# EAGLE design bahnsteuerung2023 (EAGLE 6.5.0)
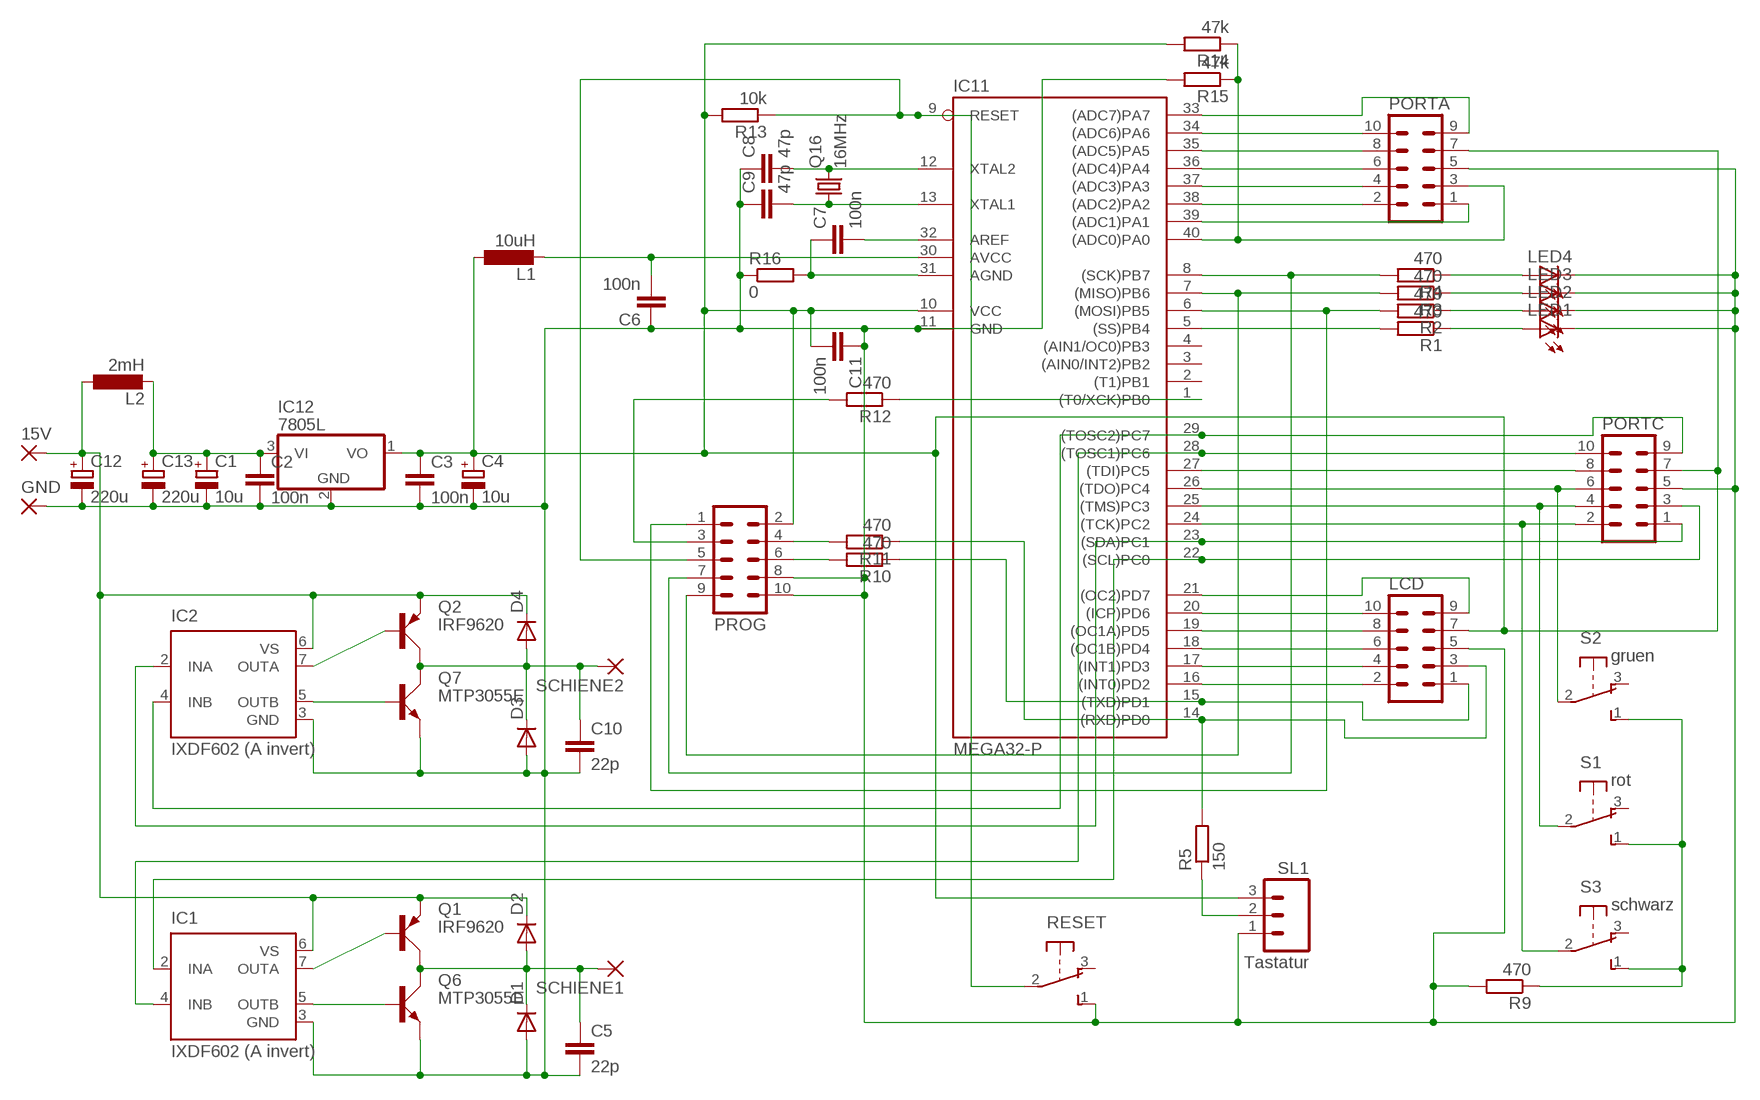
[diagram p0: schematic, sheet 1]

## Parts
15V  1,6/0,8  [1,6/0,8]
C1  10u  CPOL-EUE2.5-5  [E2,5-5]
C2  100n  C5/2.5  [C5B2.5]
C3  100n  C5/2.5  [C5B2.5]
C4  10u  CPOL-EUE2.5-5  [E2,5-5]
C5  22p  C2.5/2  [C2.5-2]
C6  100n  C5/2.5  [C5B2.5]
C7  100n  C2.5/2  [C2.5-2]
C8  47p  C2.5/2  [C2.5-2]
C9  47p  C2.5/2  [C2.5-2]
C10  22p  C2.5/2  [C2.5-2]
C11  100n  C2.5/2  [C2.5-2]
C12  220u  CPOL-EUE2.5-5  [E2,5-5]
C13  220u  CPOL-EUE2.5-5  [E2,5-5]
D1  1N4148DO35-10  [DO35-10]
D2  1N4148DO35-10  [DO35-10]
D3  1N4148DO35-10  [DO35-10]
D4  1N4148DO35-10  [DO35-10]
GND  1,6/0,8  [1,6/0,8]
IC1  IXDF602 (A invert)  IR4427S  [SO08]
IC2  IXDF602 (A invert)  IR4427S  [SO08]
IC11  MEGA32-P  [DIL40]
IC12  7805L  [TO92]
L1  10uH  L-EU0204/7  [0204/7@1]
L2  2mH  L-EU0204/7  [0204/7@1]
LCD  ML10  [ML10]
LED1  LED3MM  [LED3MM]
LED2  LED3MM  [LED3MM]
LED3  LED3MM  [LED3MM]
LED4  LED3MM  [LED3MM]
PORTA  ML10  [ML10]
PORTC  ML10  [ML10]
PROG  ML10  [ML10]
Q1  IRF9620  MJE2955  [TO220AV@1]
Q2  IRF9620  MJE2955  [TO220AV@1]
Q6  MTP3055E  MJE3055  [TO220AV]
Q7  MTP3055E  MJE3055  [TO220AV]
Q16  16MHz  CRYTALHC49U-V  [HC49U-V]
R1  470  R-EU_0204/7  [0204/7]
R2  470  R-EU_0204/7  [0204/7]
R3  470  R-EU_0204/7  [0204/7]
R4  470  R-EU_0204/7  [0204/7]
R5  150  R-EU_0204/7  [0204/7]
R9  470  R-EU_0204/7  [0204/7]
R10  470  R-EU_0204/7  [0204/7]
R11  470  R-EU_0204/7  [0204/7]
R12  470  R-EU_0204/7  [0204/7]
R13  10k  R-EU_0204/7  [0204/7]
R14  47k  R-EU_0204/7  [0204/7]
R15  47k  R-EU_0204/7  [0204/7]
R16  0  R-EU_0204/2V  [0204V]
RESET  9077-1  [9077-1]
S1  rot  9077-1  [9077-1]
S2  gruen  9077-1  [9077-1]
S3  schwarz  9077-1  [9077-1]
SCHIENE1  1,6/0,8  [1,6/0,8]
SCHIENE2  1,6/0,8  [1,6/0,8]
SL1  Tastatur  M03  [03P]

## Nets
AGND [mitteldick]: C7.1 IC11.31(AGND) R16.2
AREF [mitteldick]: C7.2 IC11.32(AREF)
AVCC [mitteldick]: C6.2 IC11.30(AVCC) L1.2
GND [mitteldick]: C1.- C2.2 C3.2 C4.- C5.2 C6.1 C8.1 C9.1 C10.2 C11.1 C12.- C13.- D1.A D3.A GND.1(P) IC1.3(GND) IC2.3(GND) IC11.11(GND) IC12.2(GND) LCD.5 LED1.K(C) LED2.K(C) LED3.K(C) LED4.K(C) PORTA.5 PORTC.5 PROG.8 PROG.10 Q6.E Q7.E R9.2 R15.2 R16.1 RESET.1(S) SL1.1
N$1: IC1.2(INA) IC11.22((SCL)PC0) PORTC.3
N$2: IC2.2(INA) IC11.23((SDA)PC1) PORTC.1
N$3: IC11.24((TCK)PC2) PORTC.2 S3.2(P)
N$4: IC11.25((TMS)PC3) PORTC.4 S1.2(P)
N$5 [mitteldick]: IC2.5(OUTB) Q7.B
N$6: IC11.5((SS)PB4) R1.2
N$7: LED1.A R1.1
N$8: LED2.A R2.1
N$9: LED3.A R3.1
N$10: LED4.A R4.1
N$11 [mitteldick]: IC11.16((INT0)PD2) LCD.2
N$12 [mitteldick]: IC11.17((INT1)PD3) LCD.4
N$13 [mitteldick]: IC11.18((OC1B)PD4) LCD.6
N$14 [mitteldick]: IC11.19((OC1A)PD5) LCD.8
N$15 [mitteldick]: IC11.20((ICP)PD6) LCD.10
N$16 [mitteldick]: IC11.21((OC2)PD7) LCD.9
N$17 [mitteldick]: IC1.5(OUTB) Q6.B
N$18 [mitteldick]: IC11.26((TDO)PC4) PORTC.6 S2.2(P)
N$19 [mitteldick]: IC11.27((TDI)PC5) PORTC.8
N$20 [mitteldick]: IC1.4(INB) IC11.28((TOSC1)PC6) PORTC.10
N$21 [mitteldick]: IC2.4(INB) IC11.29((TOSC2)PC7) PORTC.9
N$22 [mitteldick]: IC11.39((ADC1)PA1) PORTA.1
N$23 [mitteldick]: IC11.38((ADC2)PA2) PORTA.2
N$24 [mitteldick]: IC11.37((ADC3)PA3) PORTA.4
N$25 [mitteldick]: IC11.36((ADC4)PA4) PORTA.6
N$26 [mitteldick]: IC11.35((ADC5)PA5) PORTA.8
N$27 [mitteldick]: IC11.34((ADC6)PA6) PORTA.10
N$28 [mitteldick]: IC11.33((ADC7)PA7) PORTA.9
N$29 [mitteldick]: R9.1 S1.1(S) S2.1(S) S3.1(S)
N$30: R5.1 SL1.2
N$31 [mitteldick]: C1.+ C2.1 C13.+ IC12.3(VI) L2.2
N$32: C5.1 D1.C D2.A Q1.C Q6.C SCHIENE1.1(P)
N$34: IC1.7(OUTA) Q1.B
N$35: C10.1 D3.C D4.A Q2.C Q7.C SCHIENE2.1(P)
N$37: IC2.7(OUTA) Q2.B
N$122: IC11.40((ADC0)PA0) PORTA.3 R14.1 R15.1
N$135: IC11.6((MOSI)PB5) PROG.1 R2.2
N$136: IC11.7((MISO)PB6) PROG.9 R3.2
N$147: IC11.14((RXD)PD0) LCD.3 R5.2 R11.1
N$150: IC11.1((T0/XCK)PB0) R12.1
N$152: C8.2 IC11.12(XTAL2) Q16.2
N$153: C9.2 IC11.13(XTAL1) Q16.1
N$156: IC11.9(RESET) PROG.5 R13.1 RESET.2(P)
N$157: PROG.4 R11.2
N$158: PROG.6 R10.2
N$159: PROG.3 R12.2
N$161: IC11.15((TXD)PD1) LCD.1 R10.1
N$170: IC11.8((SCK)PB7) PROG.7 R4.2
VCC [mitteldick]: C3.1 C4.+ C11.2 IC11.10(VCC) IC12.1(VO) L1.1 LCD.7 PORTA.7 PORTC.7 PROG.2 R13.2 R14.2 SL1.3
VS [mitteldick]: 15V.1(P) C12.+ D2.C D4.C IC1.6(VS) IC2.6(VS) L2.1 Q1.E Q2.E
Unconnected: IC11.2((T1)PB1) IC11.3((AIN0/INT2)PB2) IC11.4((AIN1/OC0)PB3) RESET.3(O) S1.3(O) S2.3(O) S3.3(O)

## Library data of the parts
15V GND SCHIENE1 SCHIENE2 = wirepad:1,6/0,8: THROUGH-HOLE PAD
C1 C4 C12 C13 = rcl:CPOL-EU: POLARIZED CAPACITOR, European symbol
C2 C3 C5-C11 = capacitor-wima:C: CAPACITOR
D1-D4 = diode:1N4148: DIODE
IC1 IC2 = ir:IR4427: DUAL LOW SIDE DRIVER Source: ID4426.pdf; MF: INTERNATIONAL RECTIFIER(IR); MPN: IR4427STRPBF; OC_FARNELL: 8639094; OC_NEWARK: 63J7933
IC11 = atmel:MEGA32-P: MICROCONTROLLER 32 Kbytes FLASH 2 Kbytes SRAM 1 Kbytes EEPROM USART 8-channel 10 bit ADC Source: www.atmel.com .. doc2503.pdf
IC12 = linear:78*: Positive VOLTAGE REGULATOR Source: http://cache.national.com/ds/LM/LM78L05.pdf http://www.fairchildsemi.com/ds/LM/LM7805.pdf
L1 L2 = rcl:L-EU: INDUCTOR, European symbol
LCD PORTA PORTC PROG = con-harting-ml:ML10: HARTING
LED1-LED4 = led:LED: LED
Q1 Q2 = transistor-power:MJE2955: PNP TRANSISTOR
Q6 Q7 = transistor-power:MJE3055: NPN TRANSISTOR
Q16 = crystal:CRYTAL: CRYSTAL
R1-R5 R9-R16 = rcl:R-EU_: RESISTOR, European symbol
RESET S1-S3 = switch-misc:9077-1: MARQUARDT SWITCH
SL1 = con-amp-quick:M03: AMP QUICK CONNECTOR; OC_FARNELL: unknown; OC_NEWARK: unknown

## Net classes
1 dick: width 1.016 mm, clearance 0.61 mm
2 mitteldick: width 0.762 mm

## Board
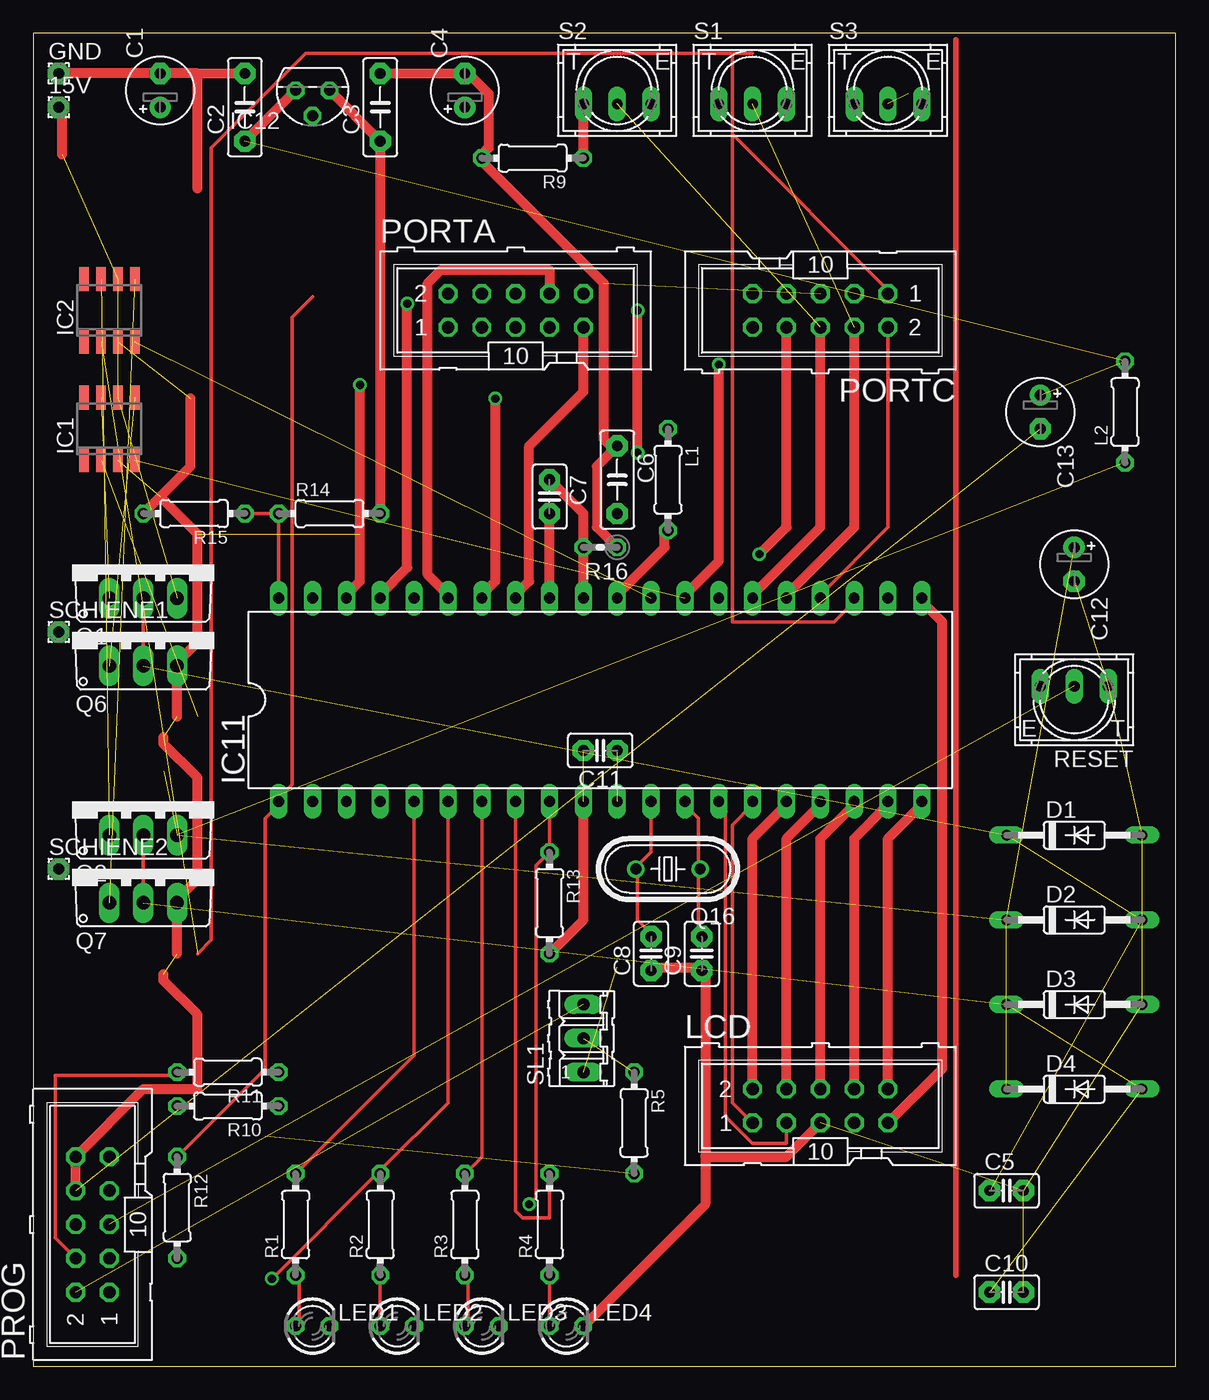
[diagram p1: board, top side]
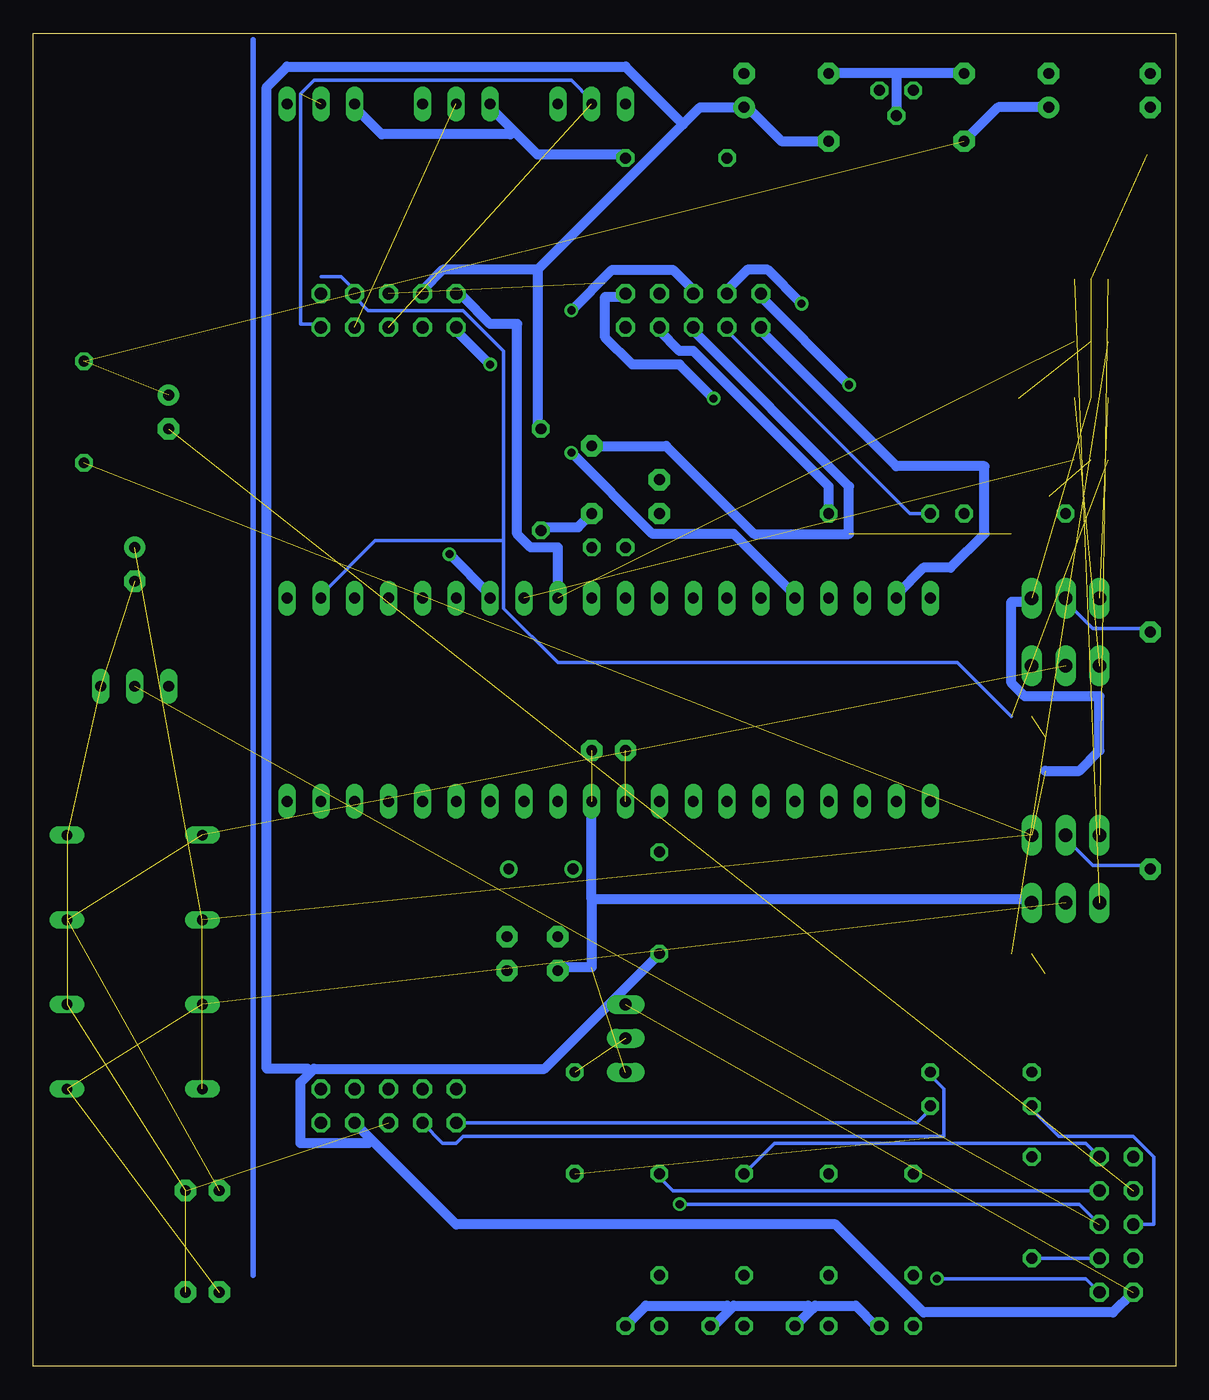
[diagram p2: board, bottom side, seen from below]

Size 85.7 x 100 mm. Coordinates in mm from the lower left corner, seen from the top.
Outline: 0,0 85.7,0 85.7,100 0,100 0,0
Copper layers (1*16): Top 0.035mm / dielectric 1.5mm / Bottom 0.035mm
Design rules "default": minimum track width 10mil, minimum drill 24mil, track to track 8mil, track to pad 8mil, pad to pad 8mil, via to via 8mil, smd to smd 8mil, copper to edge 40mil, drill to drill 8mil, minimum pad ring 10mil, minimum via ring 8mil, stop-mask expansion 4mil, vias tented up to drill 0mil, thermal gap 10mil

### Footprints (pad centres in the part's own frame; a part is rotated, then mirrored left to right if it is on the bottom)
1,6/0,8 = drill 0.813 pad 1.6 octagon: 1 0,0
E2,5-5 = drill 0.813 pad 1.6: + -1.27,0 | drill 0.813 pad 1.6 octagon: - 1.27,0
C5B2.5 = drill 0.813 pad 1.6 octagon: 1 -2.54,0; 2 2.54,0
C2.5-2 = drill 0.813 pad 1.6 octagon: 1 -1.27,0; 2 1.27,0
DO35-10 = drill 0.813 long: A 5.08,0; C -5.08,0
SO08 = smd 0.72 x 1.78: 1 -1.905,-2.35; 2 -0.635,-2.35; 3 0.635,-2.35; 4 1.905,-2.35; 5 1.905,2.35; 6 0.635,2.35; 7 -0.635,2.35; 8 -1.905,2.35
DIL40 = drill 0.813 long: 1 -24.13,-7.62; 2 -21.59,-7.62; 3 -19.05,-7.62; 4 -16.51,-7.62; 5 -13.97,-7.62; 6 -11.43,-7.62; 7 -8.89,-7.62; 8 -6.35,-7.62; 9 -3.81,-7.62; 10 -1.27,-7.62; 11 1.27,-7.62; 12 3.81,-7.62; 13 6.35,-7.62; 14 8.89,-7.62; 15 11.43,-7.62; 16 13.97,-7.62; 17 16.51,-7.62; 18 19.05,-7.62; 19 21.59,-7.62; 20 24.13,-7.62; 21 24.13,7.62; 22 21.59,7.62; 23 19.05,7.62; 24 16.51,7.62; 25 13.97,7.62; 26 11.43,7.62; 27 8.89,7.62; 28 6.35,7.62; 29 3.81,7.62; 30 1.27,7.62; 31 -1.27,7.62; 32 -3.81,7.62; 33 -6.35,7.62; 34 -8.89,7.62; 35 -11.43,7.62; 36 -13.97,7.62; 37 -16.51,7.62; 38 -19.05,7.62; 39 -21.59,7.62; 40 -24.13,7.62
TO92 = drill 0.813 octagon: 1 -1.27,0; 2 0,1.905; 3 1.27,0
0204/7@1 = drill 0.813 octagon: 1 -3.81,0; 2 3.81,0
ML10 = drill 0.914 octagon: 1 -5.08,-1.27; 2 -5.08,1.27; 3 -2.54,-1.27; 4 -2.54,1.27; 5 0,-1.27; 6 0,1.27; 7 2.54,-1.27; 8 2.54,1.27; 9 5.08,-1.27; 10 5.08,1.27
LED3MM = drill 0.813 octagon: A -1.27,0; K 1.27,0
TO220AV@1 = drill 1.016 long: B -2.54,-2.54; C 0,-2.54; E 2.54,-2.54
TO220AV = drill 1.016 long: B -2.54,-2.54; C 0,-2.54; E 2.54,-2.54
HC49U-V = drill 0.813: 1 -2.413,0; 2 2.413,0
0204/7 = drill 0.813 octagon: 1 -3.81,0; 2 3.81,0
0204V = drill 0.813 octagon: 1 -1.27,0; 2 1.27,0
9077-1 = drill 0.813 long: 1 -2.54,-1.016; 2 0,-1.016; 3 2.54,-1.016
03P = drill 0.914 long: 1 -2.54,0; 2 0,0; 3 2.54,0

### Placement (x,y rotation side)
15V  1.9,94.45 0 top
C1  9.52,95.72 90 top
C2  15.87,94.45 90 top
C3  26.03,94.45 90 top
C4  32.38,95.72 90 top
C5  73.02,13.17 0 top
C6  43.81,66.51 270 top
C7  38.73,65.24 270 top
C8  46.35,30.95 90 top
C9  50.16,30.95 90 top
C10  73.02,5.55 0 top
C11  42.54,46.19 180 top
C12  78.1,60.16 270 top
C13  75.56,71.59 270 top
D1  78.1,39.84 0 top
D2  78.1,33.49 0 top
D3  78.1,27.14 0 top
D4  78.1,20.79 0 top
GND  1.9,96.99 0 top
IC1  5.71,70.32 0 top
IC2  5.71,79.21 0 top
IC11  42.54,50 0 top
IC12  20.95,95.72 180 top
L1  47.62,66.51 270 top
L2  81.91,71.59 90 top
LCD  59.05,19.52 0 top
LED1  20.95,3.01 0 top
LED2  27.3,3.01 0 top
LED3  33.65,3.01 0 top
LED4  40,3.01 0 top
PORTA  36.19,79.21 0 top
PORTC  59.05,79.21 180 top
PROG  4.44,10.63 90 top
Q1  8.25,60.16 0 top
Q2  8.25,42.38 0 top
Q6  8.25,55.08 0 top
Q7  8.25,37.3 0 top
Q16  47.62,37.3 180 top
R1  19.68,10.63 90 top
R2  26.03,10.63 90 top
R3  32.38,10.63 90 top
R4  38.73,10.63 90 top
R5  45.08,18.25 270 top
R9  37.46,90.64 180 top
R10  14.6,19.52 180 top
R11  14.6,22.06 180 top
R12  10.79,11.9 270 top
R13  38.73,34.76 270 top
R14  22.22,63.97 0 top
R15  12.06,63.97 180 top
R16  42.54,61.43 180 top
RESET  78.1,50 180 top
S1  53.97,95.72 0 top
S2  43.81,95.72 0 top
S3  64.13,95.72 0 top
SCHIENE1  1.9,55.08 0 top
SCHIENE2  1.9,37.3 0 top
SL1  41.27,24.6 90 top

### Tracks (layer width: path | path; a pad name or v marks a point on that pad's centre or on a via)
AGND
  Top 0.762: IC11.31 R16.2 41.27,63.97 C7.1
AREF
  Top 0.762: IC11.32 C7.2
AVCC
  Top 0.762: IC11.30 43.81,57.87 47.37,61.43 47.37,62.45 L1.2
  Bottom 0.762: C6.2 44.83,62.95 47.37,62.95 L1.2
GND  (15 unrouted)
  Top 0.762: R16.1 42.29,62.95 42.29,67.53 C6.1 43.3,69.05 42.79,69.56 42.79,81.24 33.65,90.39 R9.2 33.65,90.89 34.16,91.4 34.16,95.47 32.63,96.99 C4.- C3.2 | GND.1 C1.- 12.31,96.99 | 12.31,96.99 C2.2 | LCD.5 56.51,15.71 50.41,15.71 | 50.41,15.71 50.41,29.43 C9.1 49.91,29.93 46.35,29.93 C8.1 | LED4.K 50.41,12.15 50.41,15.71 | PROG.8 PROG.10 8.25,20.79 12.31,20.79 12.31,26.38 9.77,28.92 9.77,29.43 | 10.79,30.95 Q7.E 10.79,35.01 12.31,36.54 12.31,44.16 9.77,46.7 9.77,47.21 | 10.79,48.73 Q6.E 10.79,52.79 12.31,54.32 12.31,62.45 9.52,65.24 | 9.52,65.24 11.81,67.53 11.81,72.61 | 9.52,65.24 R15.2 | 12.31,88.35 12.31,96.99
  Bottom 0.762: C6.1 38.22,69.05 31.62,62.45 24.51,62.45 24.51,66 36.19,77.69 PORTA.5 | C2.2 20.95,96.99 | 20.95,96.99 IC12.2 | 20.95,96.99 C3.2 | 27.3,4.28 LED2.K | 27.3,4.28 27.05,4.53 24,4.53 22.47,3.01 LED1.K | 33.4,4.28 33.14,4.53 27.55,4.53 27.3,4.28 | 33.4,4.28 34.67,3.01 LED3.K | LED4.K 39.75,4.53 33.65,4.53 33.4,4.28 | 43.81,35.01 43.81,29.93 46.35,29.93 C8.1 | 43.81,35.01 IC11.11 | 43.81,35.01 10.79,35.01 Q7.E
N$1  (1 unrouted)
  Bottom 0.254: 64.13,81.75 62.61,81.75 61.59,80.73 PORTC.3 61.59,80.23 60.57,79.21 53.46,79.21 50.41,76.16 50.41,61.94 | 12.31,48.73 16.38,52.79 46.35,52.79 50.41,56.86 50.41,61.94 | 50.41,61.94 60.07,61.94 64.13,57.87 IC11.22
N$2  (1 unrouted)
  Top 0.254: 12.31,30.95 13.33,31.97 13.33,91.4 20.44,98.51 52.45,98.51 | 52.45,98.51 53.97,98.51 | 52.45,98.51 52.45,92.42 | 52.45,92.42 52.45,55.84 60.07,55.84 61.59,57.37 IC11.23 | 52.45,92.42 64.13,80.73 PORTC.1
N$3  (1 unrouted)
  Top 0.254: IC11.24 59.05,57.87 64.13,62.95 PORTC.2
  Bottom 0.254: 43.81,94.96 45.33,96.48 64.64,96.48 65.65,95.47 65.65,78.19 64.13,78.19 PORTC.2
N$4  (1 unrouted)
  Top 0.762: IC11.25 56.51,57.87 61.59,62.95 PORTC.4
N$5  (1 unrouted)
N$6
  Top 0.254: R1.2 28.57,23.33 IC11.5
N$7
  Top 0.254: LED1.A 19.93,3.01 19.93,6.57 R1.1
N$8
  Top 0.254: LED2.A R2.1
N$9
  Top 0.254: LED3.A 32.63,3.01 32.63,6.57 R3.1
N$10
  Top 0.254: LED4.A R4.1
N$11
  Top 0.762: LCD.2 53.97,39.59 56.51,42.13 IC11.16
N$12
  Top 0.762: LCD.4 56.51,39.59 59.05,42.13 IC11.17
N$13
  Top 0.762: LCD.6 59.05,39.59 61.59,42.13 IC11.18
N$14
  Top 0.762: LCD.8 61.59,39.59 64.13,42.13 IC11.19
N$15
  Top 0.762: LCD.10 64.13,39.59 66.67,42.13 IC11.20
N$16
  Top 0.762: LCD.9 68.19,22.31 68.19,55.84 66.67,57.37 IC11.21
N$17  (1 unrouted)
N$18  (1 unrouted)
  Top 0.762: IC11.26 53.97,57.87 59.05,62.95 PORTC.6
N$19  (via drill 0.61)
  Top 0.762: v54.48,60.92 56.51,62.95 PORTC.8
  Bottom 0.762: v54.48,60.92 51.43,57.87 IC11.27
N$20  (via drill 0.61)  (1 unrouted)
  Top 0.762: v51.43,75.15 51.43,60.41 48.89,57.87 IC11.28
  Bottom 0.762: v51.43,75.15 53.97,77.69 PORTC.10
N$21  (1 unrouted)
  Bottom 0.762: IC11.29 46.35,61.43 48.38,61.43 49.4,62.45 49.4,78.19 51.43,78.19 53.46,80.23 53.97,80.23 PORTC.9
N$22
  Bottom 0.762: IC11.39 20.95,57.87 18.92,59.91 16.89,59.91 14.35,62.45 14.35,67.53 20.95,67.53 31.11,77.69 PORTA.1
N$23  (via drill 0.61)
  Top 0.762: v24.51,73.62 24.51,58.89 23.49,57.87 IC11.38
  Bottom 0.762: v24.51,73.62 31.11,80.23 PORTA.2
N$24  (via drill 0.61)
  Top 0.762: v28.06,79.72 28.06,59.91 26.03,57.87 IC11.37
  Bottom 0.762: v28.06,79.72 30.6,82.26 32.13,82.26 33.65,80.73 PORTA.4
N$25  (via drill 0.61)
  Top 0.762: v45.33,68.54 v45.33,79.21
  Bottom 0.762: v45.33,68.54 39.24,62.45 33.14,62.45 28.57,57.87 IC11.36 | v45.33,79.21 42.29,82.26 37.71,82.26 36.19,80.73 PORTA.6
N$26
  Top 0.762: IC11.35 31.11,57.87 29.59,59.4 29.59,81.24 30.6,82.26 38.73,82.26 PORTA.8
N$27  (via drill 0.61)
  Top 0.762: v34.67,72.61 34.67,58.89 33.65,57.87 IC11.34
  Bottom 0.762: v34.67,72.61 37.21,75.15 40.76,75.15 42.79,77.18 42.79,80.23 41.27,80.23 PORTA.10
N$28
  Top 0.762: IC11.33 36.19,57.87 37.21,58.89 37.21,69.05 41.27,73.11 PORTA.9
N$29
  Top 0.762: R9.1 S2.1
  Bottom 0.762: 49.65,92.67 47.87,90.89 41.27,90.89 R9.1 | 49.65,92.67 51.43,94.45 S1.1 | S3.1 61.59,94.45 59.56,92.42 49.91,92.42 49.65,92.67
N$30  (1 unrouted)
N$31  (2 unrouted)
  Top 0.762: C2.1 IC12.3
  Bottom 0.762: C2.1 13.33,94.45 C1.+
N$32  (3 unrouted)
  Top 0.254: Q1.C Q6.C
  Bottom 0.254: SCHIENE1.1 2.15,55.33 6.22,55.33 8.25,57.37 Q1.C
N$33
  Bottom 0.406: 69.21,6.82 69.21,99.53
N$34  (1 unrouted)
  Top 0.254: Q1.B 5.71,58.89
N$35  (3 unrouted)
  Top 0.254: Q2.C Q7.C
  Bottom 0.254: SCHIENE2.1 2.15,37.55 6.22,37.55 8.25,39.59 Q2.C
N$36
  Top 0.406: 69.21,6.82 69.21,99.53
N$37  (1 unrouted)
  Top 0.254: Q2.B 5.71,41.11
N$122
  Top 0.254: R15.1 R14.1 IC11.40
  Bottom 0.254: R14.1 19.93,63.97 33.65,77.69 PORTA.3
N$135  (via drill 0.61)
  Top 0.254: 26.03,14.69 31.11,19.77 IC11.6 | v17.9,6.57 26.03,14.69 | 26.03,14.69 R2.2
  Bottom 0.254: PROG.1 6.73,6.57 v17.9,6.57
N$136
  Top 0.254: R3.2 33.65,15.71 IC11.7
  Bottom 0.254: PROG.9 6.73,16.73 30.09,16.73 R3.2
N$147  (1 unrouted)
  Top 0.254: LCD.3 56.51,16.73 53.97,16.73 51.94,18.76 51.94,41.62 51.43,42.13 IC11.14
  Bottom 0.254: LCD.3 54.99,16.73 53.97,16.73 53.46,17.23 17.39,17.23 17.39,20.79 18.41,21.81 R11.1
N$150
  Top 0.254: R12.1 17.39,22.31 17.39,41.11 18.41,42.13 IC11.1 18.41,42.63 19.43,43.65 19.43,78.7 20.95,80.23
N$152
  Top 0.254: IC11.12 46.35,38.57 45.33,37.55 Q16.2 45.33,37.05 45.33,33.49 46.35,32.47 C8.2
N$153
  Top 0.254: C9.2 49.91,32.47 49.91,37.05 Q16.1 49.91,37.55 49.91,41.11 48.89,42.13 IC11.13
N$156  (via drill 0.61)  (1 unrouted)
  Top 0.254: IC11.9 R13.1 37.71,37.55 37.71,12.66 v37.21,12.15
  Bottom 0.254: PROG.5 7.23,12.15 v37.21,12.15
N$157
  Top 0.254: PROG.4 1.65,9.61 1.65,21.81 10.79,21.81 R11.2
N$158
  Bottom 0.254: PROG.6 1.65,10.63 1.65,15.71 3.17,17.23 8.76,17.23 10.79,19.27 R10.2
N$159
  Bottom 0.254: PROG.3 R12.2
N$161
  Top 0.254: LCD.1 52.45,19.77 52.45,40.6 53.97,42.13 IC11.15
  Bottom 0.254: LCD.1 19.43,18.25 18.41,19.27 R10.1
N$170
  Top 0.254: IC11.8 36.19,11.65 36.7,11.14 38.73,11.14 R4.2
  Bottom 0.254: PROG.7 37.71,13.17 38.73,14.19 R4.2
VCC  (2 unrouted)
  Top 0.762: R14.2 C3.1 IC12.1 | R13.2 41.27,33.49 IC11.10
  Bottom 0.762: 47.87,82.26 47.87,70.57 L1.1 | 47.87,82.26 54.99,82.26 56.51,80.73 PORTC.7 | R14.2 26.03,66 36.19,76.16 37.21,76.16 38.73,77.69 PORTA.7 | C3.1 29.59,91.91 32.13,94.45 C4.+ 35.68,94.45 36.95,93.18 | 36.95,93.18 47.87,82.26 | PROG.2 4.69,4.03 18.92,4.03 25.52,10.63 53.97,10.63 60.32,16.98 | 60.32,16.98 LCD.7 | R13.2 47.37,22.31 64.64,22.31 64.89,22.06 | 64.89,22.06 65.65,21.3 65.65,16.73 60.57,16.73 60.32,16.98 | 36.95,93.18 41.27,97.5 66.67,97.5 68.19,95.97 68.19,22.31 65.15,22.31 64.89,22.06
VS  (8 unrouted)
  Top 0.762: 2.15,90.89 2.15,94.45 15V.1
  Bottom 0.762: 9.77,44.67 7.23,44.67 5.71,46.19 5.71,50.25 11.3,50.25 12.31,51.27 12.31,57.37 10.79,57.37 Q1.E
